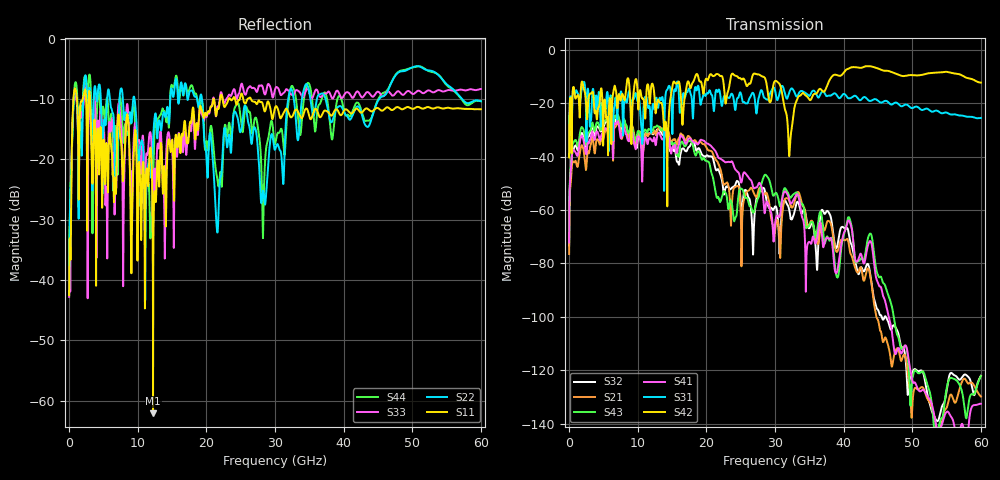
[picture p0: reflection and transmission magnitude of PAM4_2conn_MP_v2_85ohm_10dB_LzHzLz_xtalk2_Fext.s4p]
! Info: Touchstone file created by Circ.  Input file=FAB50GbE_2conn_Midplane_Examax_Topo2_v2_85ohm_10dB_LzHzLz.circ
# Hz S RI R 50
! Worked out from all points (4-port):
!   6000 points, 10 MHz to 60 GHz, reference 50 ohm
!   strongest paths, dB at 10 MHz, 15.01 GHz, 30.01 GHz, 45.01 GHz, 60 GHz:
!     S42: -40.3, -14.5, -11.7, -7.0, -12.3
!     S31: -40.0, -27.8, -15.2, -19.1, -25.6
!     S41: -72.2, -37.0, -65.3, -87.4, -132.6
!     S43: -71.4, -34.6, -53.9, -84.4, -122.3
!     S21: -76.5, -34.2, -67.8, -101.3, -129.9
!     S32: -73.4, -37.5, -58.8, -97.4, -122.1
!   lowest |S11| = -62.1 dB at 12.24 GHz (marker M1), VSWR 1.00, Z = 50 + j0.0771 ohm
!   |S11| at or under -10 dB: 3.065 GHz to 21.03 GHz (17.96 GHz wide, 149 % of centre); 21.1 GHz to 22 GHz (901.3 MHz wide, 4.18 % of centre); 26.51 GHz to end of sweep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
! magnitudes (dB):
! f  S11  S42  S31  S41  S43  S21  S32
! 10 MHz  -42.5  -40.3  -40.0  -72.2  -71.4  -76.5  -73.4
! 890 MHz  -8.2  -18.0  -16.6  -38.2  -33.8  -41.6  -36.0
! 12.24 GHz  -62.1  -13.4  -20.2  -34.3  -30.0  -31.3  -31.7
! 27.68 GHz  -10.2  -9.3  -17.6  -49.9  -54.6  -52.0  -53.7
! 32.17 GHz  -12.8  -36.6  -15.4  -56.9  -55.2  -57.4  -61.2
! 39 GHz  -11.7  -9.5  -17.0  -83.5  -85.0  -75.7  -74.1
! 60 GHz  -11.7  -12.3  -25.6  -132.6  -122.3  -129.9  -122.1
